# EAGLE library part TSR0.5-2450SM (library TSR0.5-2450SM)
4 W, 6.5 -32 VDC Vin, Single Output, 5 VDC@0.5 A DC-DC Converter Source: Datasheet
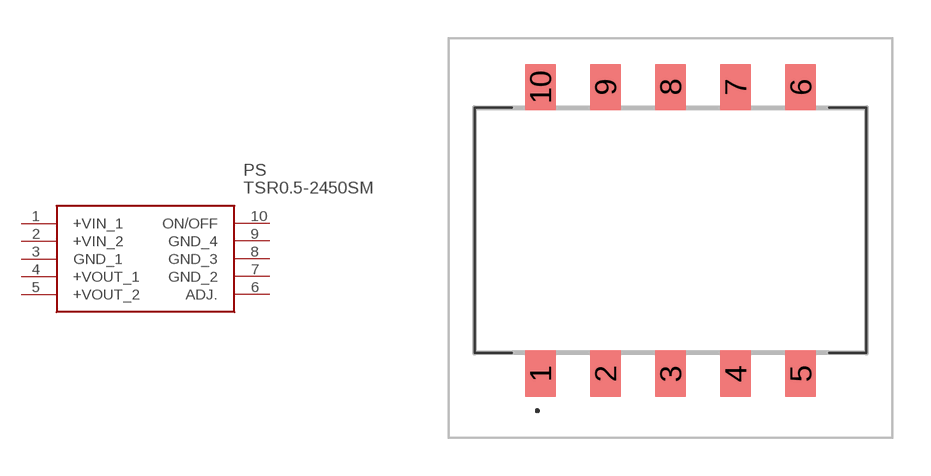
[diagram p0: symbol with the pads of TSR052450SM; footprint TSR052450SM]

Designator prefix PS

## TSR0.5-2450SM (Description: 4 W, 6.5 -32 VDC Vin, Single Output, 5 VDC@0.5 A DC-DC Converter; Height: 9.3mm; Manufacturer_Name: Traco Power; Manufacturer_Part_Number: TSR0.5-2450SM)  [TSR052450SM]
1  +VIN_1
2  +VIN_2
3  GND_1
4  +VOUT_1
5  +VOUT_2
6  ADJ.
7  GND_2
8  GND_3
9  GND_4
10  ON/OFF

## Footprint TSR052450SM (pad centres in mm)
TSR0.5-2450SM-2
smd 1.2 x 1.8: 1 -5.08,-5.6; 2 -2.54,-5.6; 3 0,-5.6; 4 2.54,-5.6; 5 5.08,-5.6; 6 5.08,5.6; 7 2.54,5.6; 8 0,5.6; 9 -2.54,5.6; 10 -5.08,5.6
